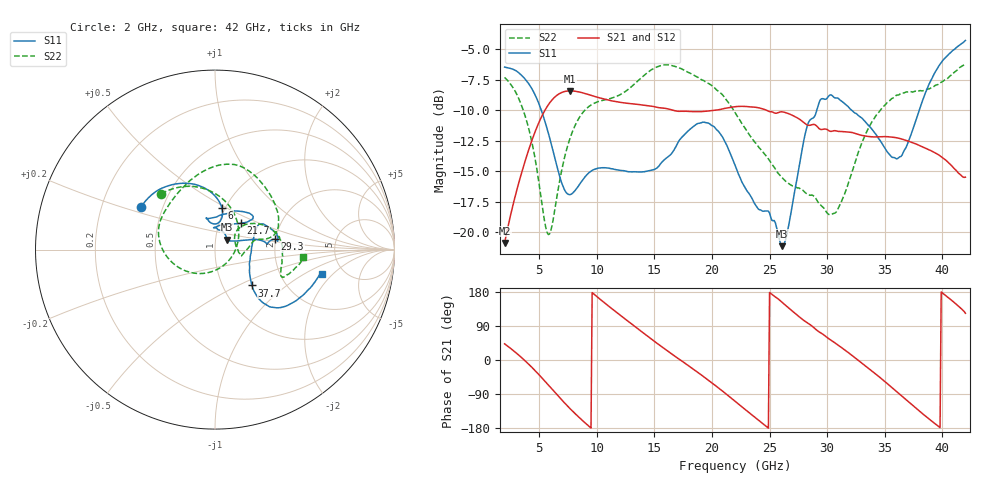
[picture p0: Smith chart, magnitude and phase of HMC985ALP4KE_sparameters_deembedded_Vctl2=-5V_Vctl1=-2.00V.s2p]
!s2p File: Measurements: S11, S21, S12, S22
# GHz S dB R 50.0
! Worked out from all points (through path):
!   401 points, 2 GHz to 42 GHz, reference 50 ohm
!   highest |S21| = -8.40 dB at 7.7 GHz (marker M1); lowest = -20.9 dB at 2 GHz (marker M2)
!   lowest |S11| = -21.1 dB at 26.1 GHz (marker M3), VSWR 1.19, Z = 56.9 + j6.32 ohm
!   |S11| at or under -10 dB: 5.188 GHz to 29.1 GHz (23.91 GHz wide, 139 % of centre); 32.14 GHz to 37.99 GHz (5.847 GHz wide, 16.7 % of centre)
!   |S22| runs from -20.2 to -6.2 dB; largest |S21 - S12| = 0.0004
!   S11 on the Smith chart (normalised r, x): 2 GHz: 0.38, +0.23; 6 GHz: 0.96, +0.47; 21.7 GHz: 1.27, +0.39; 29.3 GHz: 1.99, +0.26; 37.7 GHz: 1.37, -0.60; 42 GHz: 3.43, -1.52
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2  -6.45 149.8  -20.88 42.6  -20.88 42.6  -7.30 134.0
3.3  -6.98 129.1  -15.71 11.0  -15.71 11.0  -9.20 100.8
4.5  -8.45 106.6  -12.12 -23.4  -12.13 -23.4  -13.22 58.9
6  -12.57 80.7  -9.28 -73.0  -9.28 -73.0  -19.91 -64.2
7.7  -16.91 91.5  -8.40 -128.9  -8.40 -128.9  -12.23 -161.5
8.7  -15.81 102.3  -8.55 -158.1  -8.55 -158.1  -10.29 174.3
10.2  -14.74 104.9  -8.96 162.6  -8.97 162.6  -9.26 152.2
12.2  -14.94 105.3  -9.36 114.3  -9.37 114.3  -8.62 127.0
15.4  -14.56 84.9  -9.79 40.4  -9.79 40.4  -6.38 82.4
18.4  -11.32 49.7  -10.11 -24.6  -10.11 -24.6  -7.12 48.8
21.7  -13.76 45.6  -9.74 -101.3  -9.75 -101.3  -9.72 12.8
22  -14.48 49.9  -9.70 -108.8  -9.71 -108.8  -10.18 12.1
24.1  -18.15 90.4  -9.80 -160.2  -9.81 -160.2  -13.07 12.7
26.1  -21.14 38.9  -10.12 152.0  -10.13 152.0  -15.53 -3.7
28.7  -10.66 5.8  -11.17 89.2  -11.18 89.2  -16.95 -10.3
29.3  -9.37 9.7  -11.50 74.2  -11.50 74.3  -17.66 -5.3
30.8  -8.98 13.6  -11.69 42.3  -11.70 42.4  -18.33 26.1
32.4  -10.21 26.7  -11.89 6.3  -11.89 6.3  -14.36 41.4
35.4  -13.60 7.1  -12.18 -67.0  -12.18 -67.0  -9.23 16.8
37.7  -10.85 -44.2  -12.75 -126.9  -12.76 -126.8  -8.44 -6.5
39.8  -6.22 -41.3  -13.73 -178.3  -13.73 -178.2  -7.75 -22.1
42  -4.27 -13.1  -15.48 123.4  -15.49 123.5  -6.17 -4.8
